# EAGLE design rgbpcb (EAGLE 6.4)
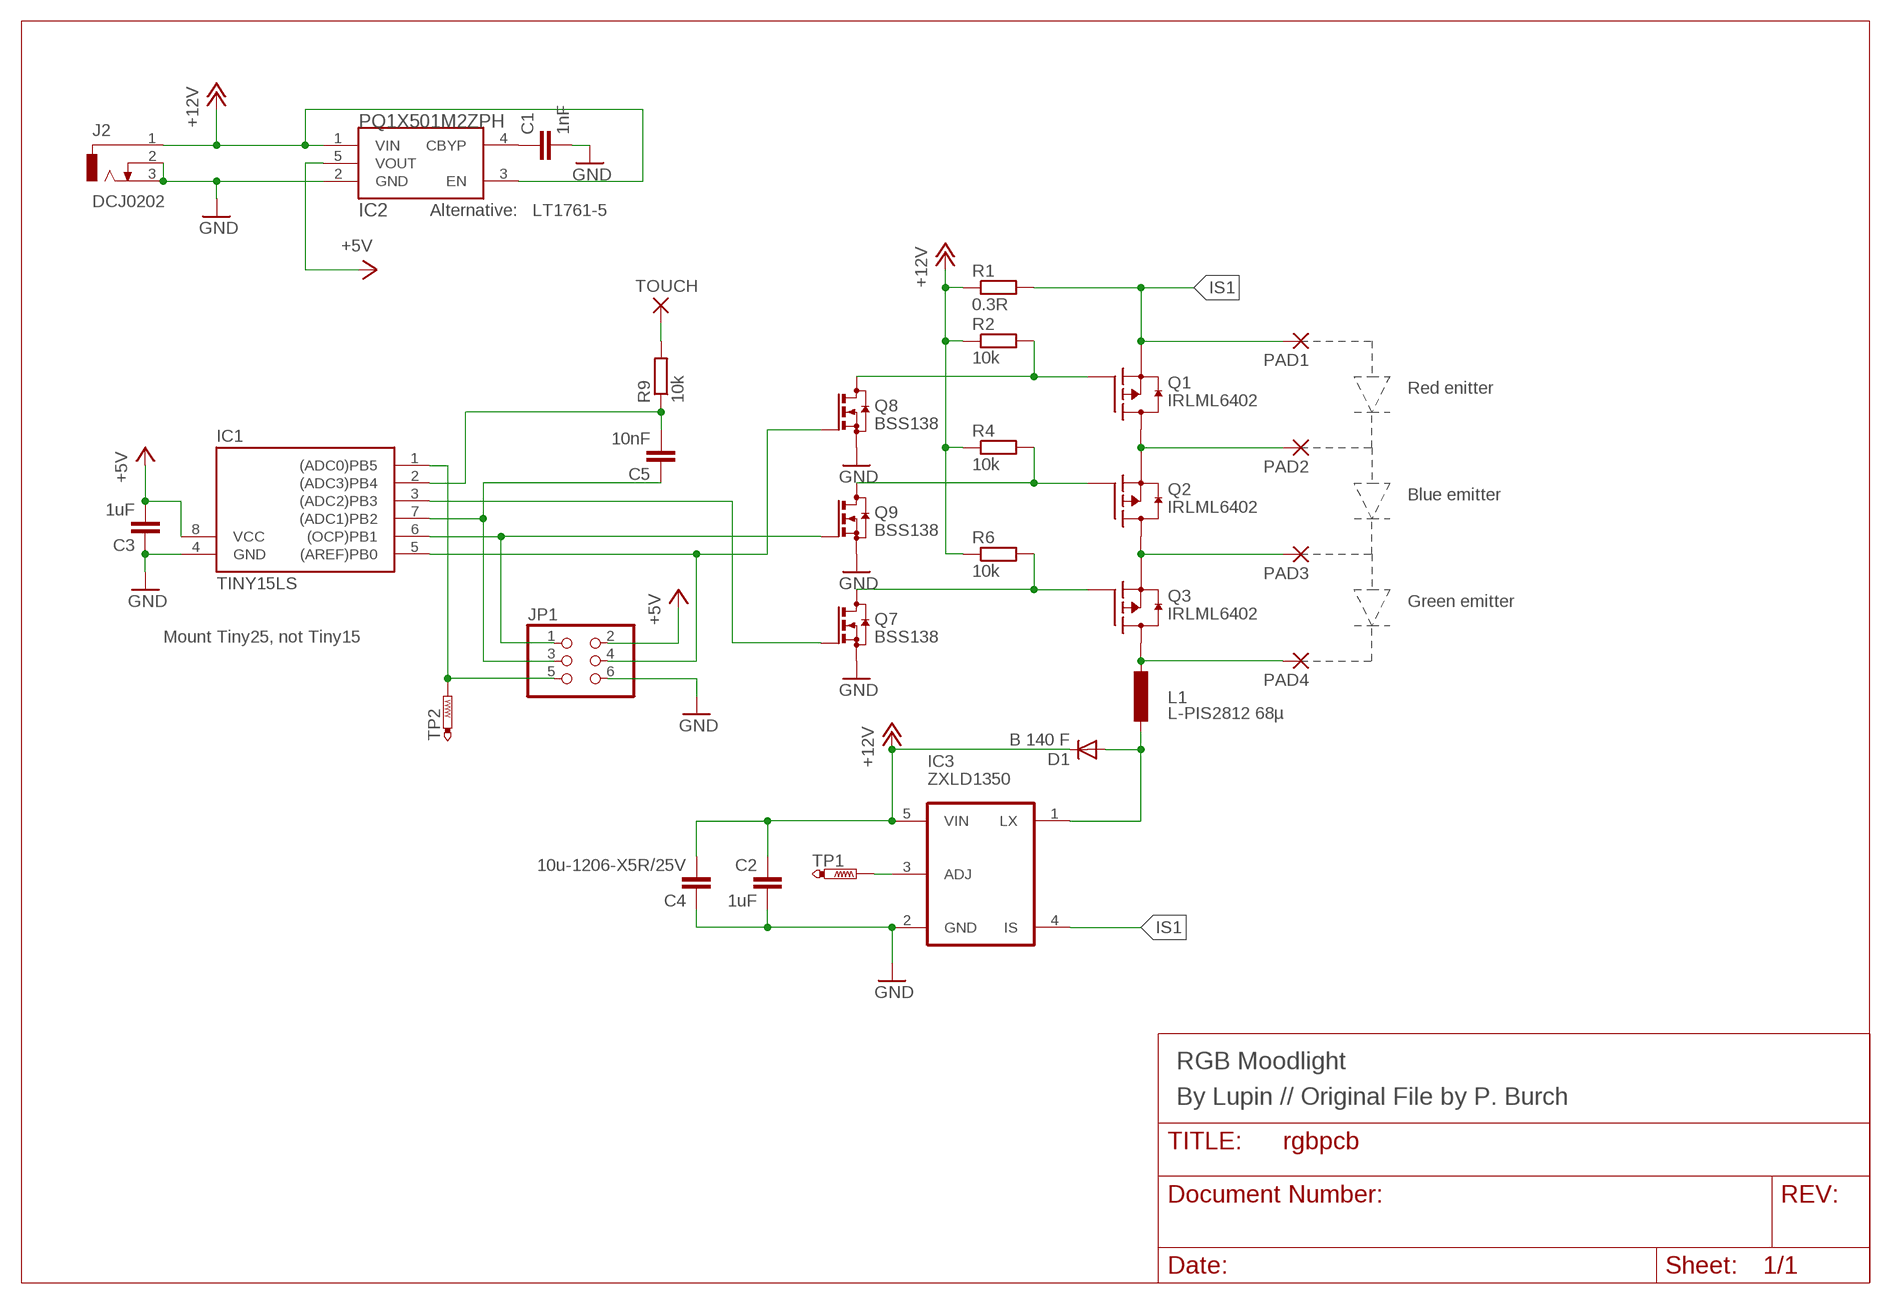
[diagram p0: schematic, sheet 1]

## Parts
C1  1nF  C-EUC0603  [C0603]
C2  1uF  C-EUC0603  [C0603]
C3  1uF  C-EUC0603  [C0603]
C4  10u-1206-X5R/25V  C-EUC1206  [C1206]
C5  10nF  C-EUC0603  [C0603]
D1  B 140 F  DIODE-DO-214AC  [DO-214AC]
IC1  TINY15LS  [SOIC8]
IC2  PQ1X501M2ZPH  IRU1205-33  [SOT23-5]
IC3  ZXLD1350  [SOT23-5]
J2  DCJ0202  [DCJ0202]
JP1  PINHD-2X3_2.54-SMD  [2X03SMD]
L1  L-PIS2812 68µ  L-EUPIS2816  [PIS2816]
PAD1  SMD2  [SMD1,27-2,54]
PAD2  SMD2  [SMD1,27-2,54]
PAD3  SMD2  [SMD1,27-2,54]
PAD4  SMD2  [SMD1,27-2,54]
Q1  IRLML6402  IRLML6302  [SOT23]
Q2  IRLML6402  IRLML6302  [SOT23]
Q3  IRLML6402  IRLML6302  [SOT23]
Q7  BSS138  BSS123  [SOT23]
Q8  BSS138  BSS123  [SOT23]
Q9  BSS138  BSS123  [SOT23]
R1  0.3R  R-EU_R1206  [R1206]
R2  10k  R-EU_R0603  [R0603]
R4  10k  R-EU_R0603  [R0603]
R6  10k  R-EU_R0603  [R0603]
R9  10k  R-EU_R0603  [R0603]
TOUCH  SMD2  [SMD1,27-2,54]
TP1  PTR1B1,27  [B1,27]
TP2  PTR1B1,27  [B1,27]

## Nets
+5V: C3.2 IC1.8(VCC) IC2.5(VOUT) JP1.2
+12V: C2.1 C4.2 D1.C IC2.1(VIN) IC2.3(EN) IC3.5(VIN) J2.1 R1.1 R2.1 R4.1 R6.1
GND: C1.2 C2.2 C3.1 C4.1 IC1.4(GND) IC2.2(GND) IC3.2(GND) J2.2 J2.3 JP1.6 Q7.2(S) Q8.2(S) Q9.2(S)
IS1: IC3.4(IS) PAD1.1(P) Q1.2(S) R1.2
N$1: Q2.1(G) Q9.3(D) R4.2
N$2: Q3.1(G) Q7.3(D) R6.2
N$3: D1.A IC3.1(LX) L1.2
N$4: C1.1 IC2.4(CBYP)
N$5: IC1.6((OCP)PB1) JP1.1 Q9.1(G)
N$7: Q1.1(G) Q8.3(D) R2.2
N$8: IC3.3(ADJ) TP1.TP
N$10: C5.1 IC1.7((ADC1)PB2) JP1.3
N$12: R9.2 TOUCH.1(P)
N$13: C5.2 IC1.2((ADC3)PB4) R9.1
N$16: IC1.1((ADC0)PB5) JP1.5 TP2.TP
OUT1: PAD2.1(P) Q1.3(D) Q2.2(S)
OUT2: PAD3.1(P) Q2.3(D) Q3.2(S)
OUT3: L1.1 PAD4.1(P) Q3.3(D)
PWM1: IC1.5((AREF)PB0) JP1.4 Q8.1(G)
PWM3: IC1.3((ADC2)PB3) Q7.1(G)

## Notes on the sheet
- Alternative:   LT1761-5
- Red enitter
- Blue emitter
- Green emitter
- Mount Tiny25, not Tiny15
- RGB Moodlight
- By Lupin // Original File by P. Burch

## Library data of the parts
C1-C5 = rcl:C-EU: CAPACITOR, European symbol
D1 = diode:DIODE-: DIODE
IC1 = atmel:TINY15L: MICROCONTROLLER 2.7 V 1 Kbytes FLASH 64 bytes EEPROM 4-channel 10 bit ADC
IC2 = iru:IRU1205-33
IC3 = zetex:ZXLD1350: 350mA LED driver with internal switch Features: Supply voltage up to 30V High efficiency up to 95% Up to 1MHz switching frequency
J2 = con-jack:DCJ0202: DC POWER JACK Source: DCJ0202.pdf
JP1 = pinheadsmd:PINHD-2X3: PIN HEADER
L1 = rcl:L-EU: INDUCTOR, European symbol
PAD1-PAD4 TOUCH = wirepad:SMD2: SMD PAD
Q1-Q3 = transistor-fet:IRLML6302: P-Channel Enhancement MOSFET (HEXFET) RDSOn = 0.6R VDS = -20V IDS = 780mA
Q7-Q9 = transistor-small-signal:BSS123: N-CHANNEL MOS FET
R1 R2 R4 R6 R9 = rcl:R-EU_: RESISTOR, European symbol
TP1 TP2 = testpad:PTR1: TEST PIN

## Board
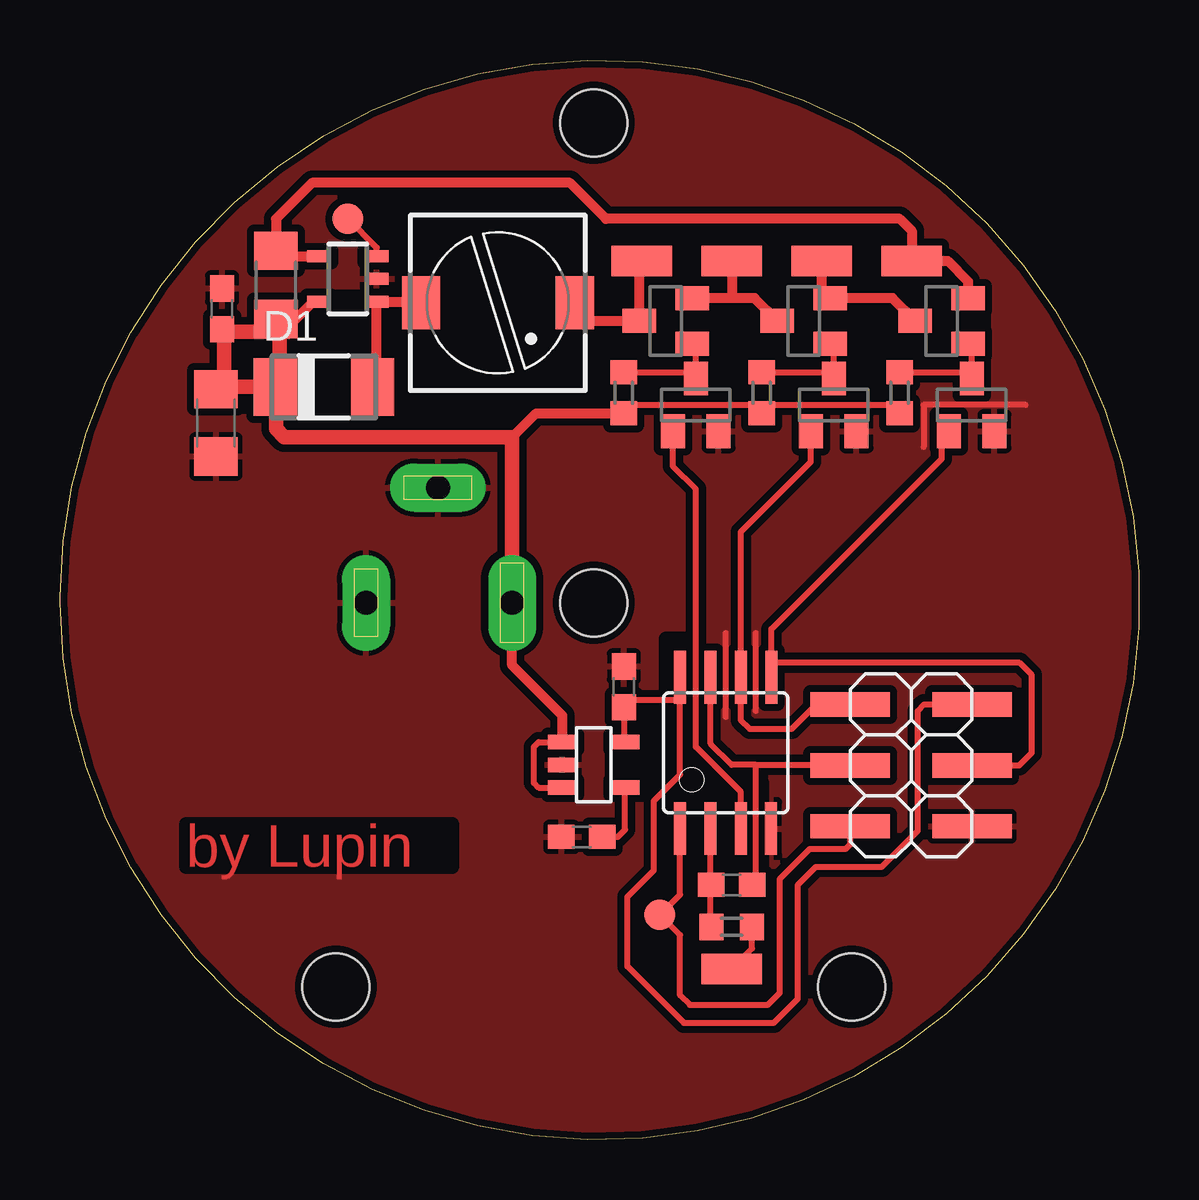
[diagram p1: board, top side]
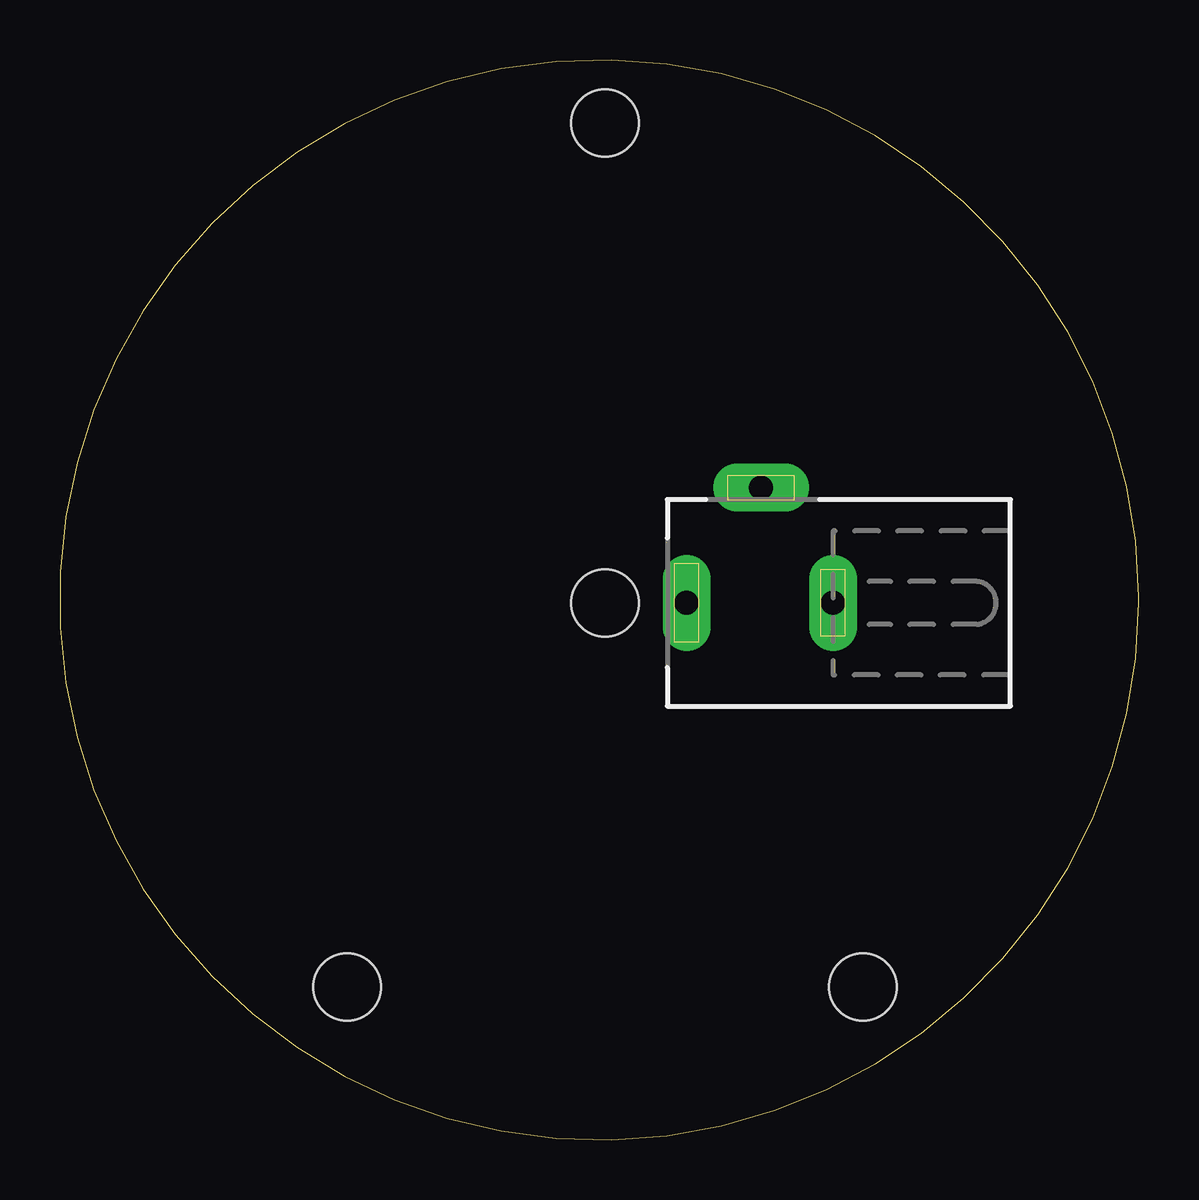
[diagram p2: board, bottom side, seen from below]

Size 44.97 x 44.99 mm. Coordinates in mm from the lower left corner, seen from the top.
Outline: 0,22.62 arc-359 0,22.37 0,22.62
Copper layers (1*16): Top 0.035mm / dielectric 1.5mm / Bottom 0.035mm
Design rules "PCB-POOL *": minimum track width 8mil, minimum drill 12mil, track to track 8mil, track to pad 8mil, pad to pad 8mil, via to via 8mil, smd to smd 0mil, copper to edge 0.1mm, drill to drill 8mil, minimum pad ring 8mil, minimum via ring 6mil, stop-mask expansion 3mil, vias tented up to drill 0mil, thermal gap 8mil
Holes 2.8 mm at 22.25,42.37 11.5,6.37 33,6.37 22.25,22.37
tRestrict: area 14.5,31.1 to 22,38.6; area 28.5,11.4 to 29.2,14.9; area 25.2,15.4 to 26.5,20.9; area 23,15.1 to 24,16.1; area 10.5,34.1 to 13.5,35.1; area 38.2,33.6 to 38.5,34.6

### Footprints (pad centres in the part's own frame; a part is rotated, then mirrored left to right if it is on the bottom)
C0603 = smd 1.1 x 1: 1 -0.85,0; 2 0.85,0
C1206 = smd 1.6 x 1.8: 1 -1.4,0; 2 1.4,0
DO-214AC = smd 1.8 x 2.4: A 2.025,0; C -2.025,0
SOIC8 = smd 0.5 x 2.2: 1 -1.905,-3.154; 2 -0.645,-3.154; 3 0.625,-3.154; 4 1.895,-3.154; 5 1.905,3.154; 6 0.635,3.154; 7 -0.635,3.154; 8 -1.905,3.154
SOT23-5 = smd 0.6 x 1.2: 1 -0.95,-1.306; 2 0,-1.306; 3 0.95,-1.306; 4 0.95,1.306; 5 -0.95,1.306
SOT23-5' = smd 0.5 x 1: 1 -0.95,-1.2; 2 0,-1.2; 3 0.95,-1.2; 4 0.95,1.2; 5 -0.95,1.2
DCJ0202 = drill 1 pad 2 long: 1 0,3.1; 2 4.8,0; 3 0,-3
2X03SMD = smd 1.016 x 3.302: 1 -1.27,-3.81; 2 -1.27,1.27; 3 1.27,-3.81; 4 1.27,1.27; 5 3.81,-3.81; 6 3.81,1.27
PIS2816 = smd 2.2 x 1.6: 1 0,3.2; 2 0,-3.2
SMD1,27-2,54 = smd 1.27 x 2.54: 1 0,0
SOT23 = smd 1 x 1.4: 1 -0.95,-1.1; 2 0.95,-1.1; 3 0,1.1
R1206 = smd 1.6 x 1.803: 1 -1.422,0; 2 1.422,0
R0603 = smd 1 x 1.1: 1 -0.85,0; 2 0.85,0
B1,27 = smd 1.27 x 1.27: TP 0,0

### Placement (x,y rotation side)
C1  21.75,12.62 180 top
C2  6.75,34.62 90 top
C3  23.5,18.87 270 top
C4  6.5,29.87 90 top
C5  28,10.62 180 top
D1  11,31.37 0 top
IC1  27.75,16.12 0 top
IC2  22.25,15.62 270 top
IC3  ZXLD1350  [SOT23-5']  12,35.87 90 top
J2  15.75,22.37 90 bottom
JP1  36.75,16.87 270 top
L1  18.25,34.87 270 top
PAD1  35.5,36.62 90 top
PAD2  31.75,36.62 90 top
PAD3  28,36.62 90 top
PAD4  24.25,36.62 270 top
Q1  36.75,34.12 90 top
Q2  31,34.12 90 top
Q3  25.25,34.12 90 top
Q7  26.5,30.62 0 top
Q8  38,30.62 0 top
Q9  32.25,30.62 0 top
R1  9,35.62 90 top
R2  35,31.12 90 top
R4  29.25,31.12 90 top
R6  23.5,31.12 90 top
R9  28,8.87 0 top
TOUCH  28,7.12 90 top
TP1  12,38.37 0 top
TP2  25,9.37 0 top

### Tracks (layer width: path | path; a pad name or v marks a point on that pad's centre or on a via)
+5V
  Top 0.254: 23.75,18.32 25.89,18.32 IC1.8 25.84,15.21 24.75,14.12 24.75,11.22 23.65,10.12 23.65,7.22 26,4.87 29.75,4.87 30.75,5.87 30.75,10.62 31.5,11.37 34.25,11.37 35.75,12.87 35.75,17.87 36.02,18.14 JP1.2 | C3.2 23.9,17.97 23.75,18.32 | IC2.5 23.44,16.56 23.5,16.62 C3.2 | 23.75,18.32 C3.2
+12V
  Top 0.254: 29.25,30.62 23.5,30.62 R6.1 | 29.25,30.62 34.9,30.62 R2.1 | 29.25,30.62 R4.1 | IC2.1 19.95,16.57 19.75,16.37 19.75,14.87 19.95,14.67 IC2.3
  Top 0.406: 9.5,33.67 R1.1 | IC2.1 20.94,17.68 18.85,19.77 J2.1 | IC3.5 10.54,34.92 9.15,33.52 | 18.85,29.27 19.85,30.27 R6.1
  Top 0.61: 6.85,33.67 9.5,33.67 | J2.1 18.85,29.27 9.35,29.27 9,29.62 9,31.34 D1.C | D1.C 6.85,31.37 | 6.85,31.37 C4.2 | 6.85,31.37 6.85,33.67 | 6.85,33.67 C2.1 | 9.15,33.52 9.15,31.54 D1.C
GND
  Top 0.254: 27.75,17.62 27.75,21.12 | 29,17.87 29,21.12 | 40.25,30.62 36,30.62 36,28.87
  pour Top (isolate 0.305): 0,45.62 45.25,45.62 45.25,-0.13 0,-0.13
IS1
  Top 0.406: R1.2 9,37.62 | IC3.4 9.72,36.82 R1.2 | R1.2 9,38.37 10.5,39.87 21.25,39.87 22.75,38.37 35,38.37 35.5,37.87 PAD1.1 37,36.62 37.85,35.77 Q1.2
N$1
  Top 0.254: R4.2 32,31.97 Q9.3 32.25,33.02 Q2.1
N$2
  Top 0.254: R6.2 26.25,31.97 Q7.3 26.5,33.02 Q3.1
N$3
  Top 0.406: L1.2 15,34.92 IC3.1 13.2,31.44 D1.A
N$4
  Top 0.254: C1.1 23.25,12.62 23.56,12.93 IC2.4
N$5
  Top 0.254: JP1.1 32.42,18.12 31.5,18.12 30.5,17.12 28.75,17.12 28.39,17.48 IC1.6 28.39,25.33 31.3,28.25 Q9.1
N$7
  Top 0.254: R2.2 37.75,31.97 Q8.3 38,33.02 Q1.1
N$8
  Top 0.254: IC3.3 13.2,37.17 TP1.TP
N$10
  Top 0.254: IC1.7 27.11,16.5 28,15.62 29,15.62 | 29,15.62 31.67,15.62 JP1.3 | C5.1 29,10.62 29,15.62
N$12
  Top 0.254: R9.2 28.85,7.97 TOUCH.1
N$13
  Top 0.254: 27.11,10.62 C5.2 | 27.11,10.62 IC1.2 | 27.11,10.62 27.11,9.16 R9.1
N$16
  Top 0.254: 25.85,12.72 25.84,12.72 IC1.1 25.84,10.21 TP2.TP 25.84,8.52 25.84,6.02 25.85,6.02 26.25,5.62 29.5,5.62 30,6.12 30,10.87 31.25,12.12 32.75,12.12 32.94,12.31 JP1.5
OUT1
  Top 0.406: Q1.3 34.7,35.07 Q2.2 31.75,35.42 PAD2.1
OUT2
  Top 0.406: 26.45,35.07 Q3.2 28,35.07 | Q2.3 28.95,35.07 28,35.07 | PAD3.1 28,35.07
OUT3
  Top 0.406: L1.1 21.5,34.37 21.75,34.12 Q3.3 24.15,36.52 PAD4.1
PWM1
  Top 0.254: IC1.5 29.66,19.87 | 29.66,19.87 29.66,21.27 36.75,28.37 36.75,29.72 Q8.1 | JP1.4 39.98,15.6 40.5,16.12 40.5,19.37 40,19.87 29.66,19.87
PWM3
  Top 0.254: IC1.3 28.38,14.49 26.5,16.37 26.5,27.12 25.55,28.07 Q7.1

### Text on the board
Top: by Lupin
